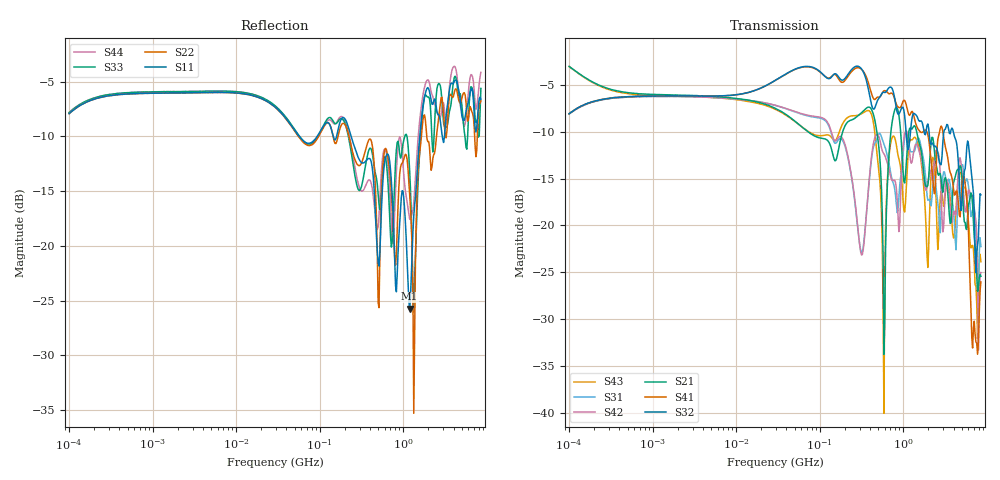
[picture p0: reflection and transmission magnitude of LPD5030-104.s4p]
# MHz S MA R 50
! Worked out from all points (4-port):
!   498 points, 100 kHz to 8.5 GHz, reference 50 ohm
!   strongest paths, dB at 100 kHz, 1.698 MHz, 29.49 MHz, 500.7 MHz, 8.5 GHz:
!     S32: -8.1, -6.2, -4.5, -6.6, -16.7
!     S41: -8.1, -6.2, -4.5, -6.3, -26.0
!     S21: -3.1, -6.1, -7.5, -11.0, -25.4
!     S42: -8.1, -6.3, -7.2, -10.4, -25.0
!     S31: -8.1, -6.3, -7.2, -10.4, -22.2
!     S43: -3.1, -6.2, -7.6, -13.5, -23.9
!   lowest |S11| = -25.7 dB at 1.192 GHz (marker M1), VSWR 1.11, Z = 46.8 - j3.86 ohm
!   |S11| at or under -10 dB: 57.02 MHz to 93.14 MHz (36.11 MHz wide, 48.1 % of centre); 237.2 MHz to 1.576 GHz (1.339 GHz wide, 148 % of centre); 2.937 GHz to 3.115 GHz (177.7 MHz wide, 5.87 % of centre)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
0.1  0.4022 34.8  0.7034 -19.3  0.3924 -143.9  0.394 36.2
     0.7034 -19.3  0.4022 34.9  0.3935 36.2  0.3923 -144.1
     0.3924 -143.9  0.3935 36.2  0.4065 34.9  0.7018 -19.6
     0.394 36.2  0.3923 -144.1  0.7018 -19.6  0.4075 35.1
70.23698  0.295 -21.0  0.3185 -109.4  0.3843 71.8  0.7004 -9.7
          0.3185 -109.4  0.2893 -22.1  0.7037 -9.6  0.3872 71.0
          0.3843 71.8  0.7037 -9.6  0.2937 -21.0  0.3203 -109.7
          0.7004 -9.7  0.3872 71.0  0.3203 -109.7  0.2923 -21.7
407.6417  0.2469 -84.5  0.4213 -28.5  0.2071 56.8  0.5219 -82.2
          0.4213 -28.5  0.3064 -81.5  0.4605 -84.4  0.2121 52.1
          0.2071 56.8  0.4605 -84.4  0.2794 -62.2  0.3988 -41.0
          0.5219 -82.2  0.2121 52.1  0.3988 -41.0  0.197 -67.4
587.4518  0.2273 -61.0  0.02056 -113.9  0.2726 -52.8  0.5218 -96.5
          0.02056 -113.9  0.2618 -63.0  0.5123 -93.9  0.2404 -55.3
          0.2726 -52.8  0.5123 -93.9  0.2468 -71.0  0.009979 59.7
          0.5218 -96.5  0.2404 -55.3  0.009979 59.7  0.2745 -64.8
1192.452  0.05162 -127.3  0.3293 -137.5  0.2576 -151.1  0.3858 171.1
          0.3293 -137.5  0.1722 170.8  0.2816 -167.4  0.2423 -155.7
          0.2576 -151.1  0.2816 -167.4  0.2214 166.1  0.282 -130.5
          0.3858 171.1  0.2423 -155.7  0.282 -130.5  0.1329 -140.2
6920.76  0.4611 -161.1  0.1055 134.2  0.1234 159.6  0.02817 157.1
         0.1055 134.2  0.3874 -164.7  0.1485 91.7  0.1338 145.2
         0.1234 159.6  0.1485 91.7  0.4909 177.6  0.0746 -179.9
         0.02817 157.1  0.1338 145.2  0.0746 -179.9  0.5605 -175.7
8500  0.4682 -28.6  0.0536 36.4  0.0772 -14.9  0.05001 78.4
      0.0536 36.4  0.4594 -38.0  0.1456 -37.1  0.05608 0.3
      0.0772 -14.9  0.1456 -37.1  0.5243 -26.9  0.06403 30.5
      0.05001 78.4  0.05608 0.3  0.06403 30.5  0.6207 -35.1
